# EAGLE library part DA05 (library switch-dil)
DIL/CODE SWITCH
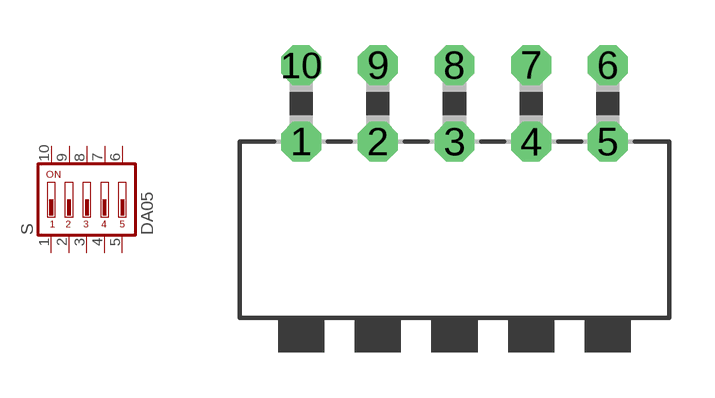
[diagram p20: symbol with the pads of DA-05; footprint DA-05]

Designator prefix S

## DA05 (MPN: MCDA05; OC_FARNELL: 1522001; OC_NEWARK: 74M2973)  [DA-05]
1  1  pas
2  2  pas
3  3  pas
4  4  pas
5  5  pas
6  6  pas
7  7  pas
8  8  pas
9  9  pas
10  10  pas

## Footprint DA-05 (pad centres in mm)
DIL/CODE SWITCH Mors distributor Buerklin, 17G586
drill 0.813 octagon: 1 -5.08,-1.27; 2 -2.54,-1.27; 3 0,-1.27; 4 2.54,-1.27; 5 5.08,-1.27; 6 5.08,1.27; 7 2.54,1.27; 8 0,1.27; 9 -2.54,1.27; 10 -5.08,1.27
